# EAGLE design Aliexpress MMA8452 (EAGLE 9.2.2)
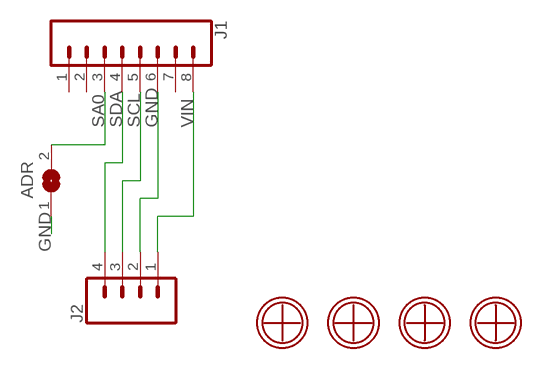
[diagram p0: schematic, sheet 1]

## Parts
ADR  SOLDERJUMPERREFLOW  [SOLDERJUMPER_REFLOW]
J1  CONN_08"  [1X08]
J2  CONN_04  [1X04]
U$1  3.2MM-5MM  [3.2MM-5MM]
U$2  3.2MM-5MM  [3.2MM-5MM]
U$3  3.2MM-5MM  [3.2MM-5MM]
U$4  3.2MM-5MM  [3.2MM-5MM]

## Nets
GND: ADR.1 J1.6 J2.2
SA0: ADR.2 J1.3
SCL: J1.5 J2.3
SDA: J1.4 J2.4
VIN: J1.8 J2.1
Unconnected: J1.1 J1.2 J1.7 U$1.P$1 U$2.P$1 U$3.P$1 U$4.P$1

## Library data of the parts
ADR = #microbuilder:SOLDERJUMPER: SMD Solder JUMPER
J1 = SparkFun-Connectors:CONN_08: Multi connection point. Often used as Generic Header-pin footprint for 0.1 inch spaced/style header connections On any of the 0.1 inch spaced packages, you can populate with these: Break Away Headers - Straight (PRT-00116) Break Away Male Headers - Right Angle (PRT-00553) Female Headers (PRT-00115)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; PROD_ID: CONN-08438
J2 = SparkFun-Connectors:CONN_04: Multi connection point. Often used as Generic Header-pin footprint for 0.1 inch spaced/style header connections On any of the 0.1 inch spaced packages, you can populate with these: Break Away Headers - Straight (PRT-00116) Break Away Male Headers - Right Angle (PRT-00553) Female Headers (PRT-00115)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; PROD_ID: CONN-09696
U$1-U$4 = #Holes:3.2MM-5MM

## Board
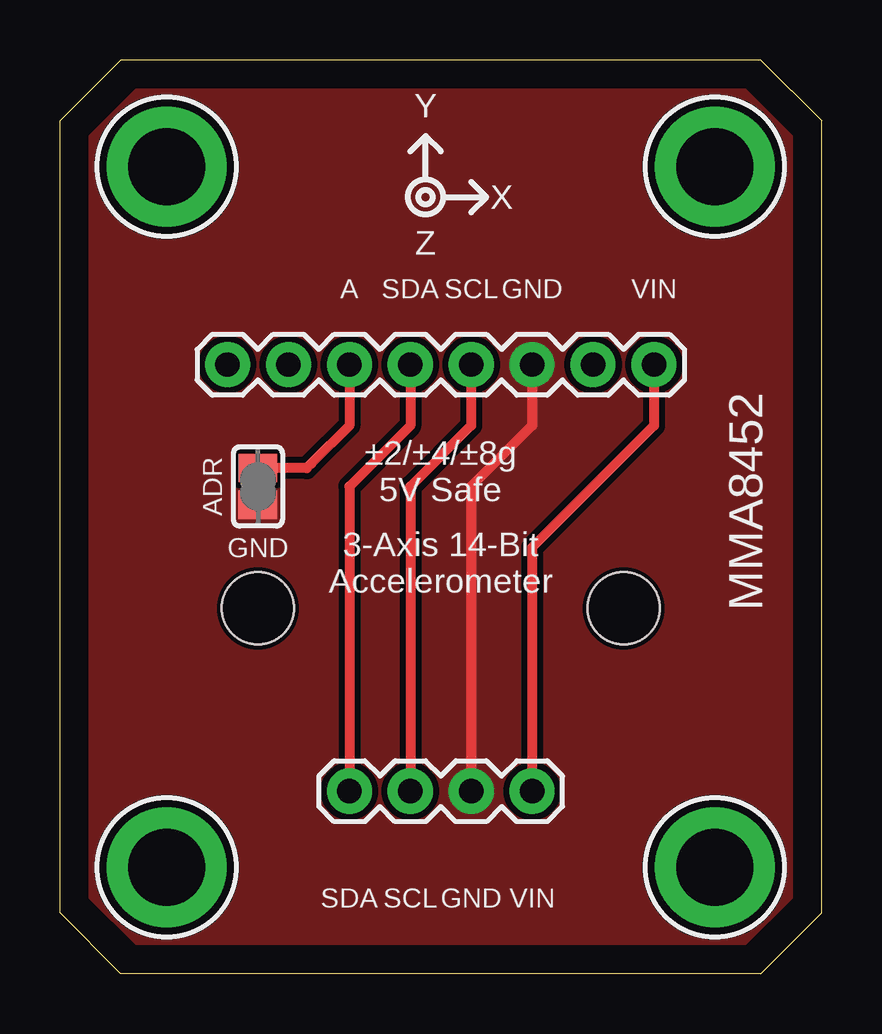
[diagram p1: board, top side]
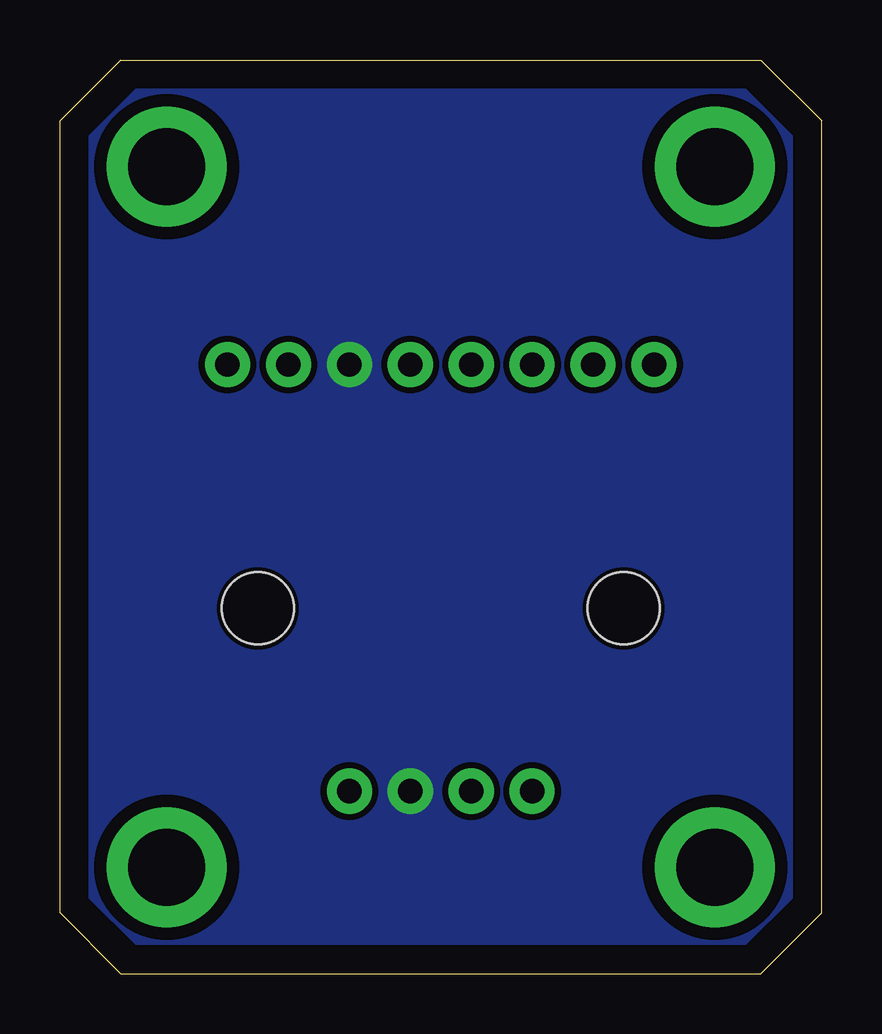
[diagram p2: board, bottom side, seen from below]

Size 31.75 x 38.1 mm. Coordinates in mm from the lower left corner, seen from the top.
Outline: 29.21,0 2.54,0 0,2.54 0,35.56 2.54,38.1 29.21,38.1 31.75,35.56 31.75,2.54 29.21,0
Copper layers (1*16): Top 0.035mm / dielectric 1.5mm / Bottom 0.035mm
Design rules "SparkFun 2 Layer Design Rule - STANDARD": minimum track width 10mil, minimum drill 20mil, track to track 10mil, track to pad 8mil, pad to pad 8mil, via to via 10mil, smd to smd 8mil, copper to edge 8mil, drill to drill 8mil, minimum pad ring 10mil, minimum via ring 10mil, stop-mask expansion 4mil, vias tented up to drill 25mil, thermal gap 10mil
Holes 3 mm at 8.25,15.24 23.5,15.24

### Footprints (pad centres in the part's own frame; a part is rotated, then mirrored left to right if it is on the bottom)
SOLDERJUMPER_REFLOW = smd 1.168 x 1.6: 1 -0.762,0; 2 0.762,0
1X08 = drill 1.016 pad 1.88: 1 0,0; 2 2.54,0; 3 5.08,0; 4 7.62,0; 5 10.16,0; 6 12.7,0; 7 15.24,0; 8 17.78,0
1X04 = drill 1.016 pad 1.88: 1 0,0; 2 2.54,0; 3 5.08,0; 4 7.62,0
3.2MM-5MM = drill 3.2 pad 5: P$1 0,0

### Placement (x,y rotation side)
ADR  8.25,20.32 90 top
J1  6.98,25.4 0 top
J2  19.69,7.62 180 top
U$1  4.45,33.66 0 top
U$2  27.3,33.66 0 top
U$3  4.45,4.45 0 top
U$4  27.3,4.45 0 top

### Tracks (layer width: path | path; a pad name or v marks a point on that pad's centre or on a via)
GND
  Top 0.406: J1.6 19.69,22.86 17.14,20.32 J2.2
  pour Bottom (no thermals): 3.18,36.83 28.57,36.83 30.48,34.92 30.48,3.17 28.57,1.27 3.18,1.27 1.27,3.17 1.27,34.92
  pour Top (no thermals): 3.18,36.83 28.57,36.83 30.48,34.92 30.48,3.17 28.57,1.27 3.18,1.27 1.27,3.17 1.27,34.92
SA0
  Top 0.406: J1.3 12.06,22.86 10.48,21.27 | 10.48,21.27 10.29,21.08 | 10.48,21.27 10.29,21.08 | 10.29,21.08 ADR.2
SCL
  Top 0.406: J2.3 14.6,20.32 17.14,22.86 J1.5
SDA
  Top 0.406: J2.4 12.06,20.32 14.6,22.86 J1.4
VIN
  Top 0.406: J1.8 24.77,22.86 19.69,17.78 J2.1

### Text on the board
tPlace: Y | X | Z | ±2/±4/±8g / 5V Safe | 3-Axis 14-Bit / Accelerometer
tNames: A | SDA | SCL | GND | VIN | ADR | MMA8452 | GND | SDA | SCL | GND | VIN

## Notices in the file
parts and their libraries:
SparkFun-Connectors: Licensing: Creative Commons ShareAlike 4.0 International - https://creativecommons.org/licenses/by-sa/4.0
This work is placed in the public domain, and may be freely used for commercial and non-commercial work with the following conditions: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
